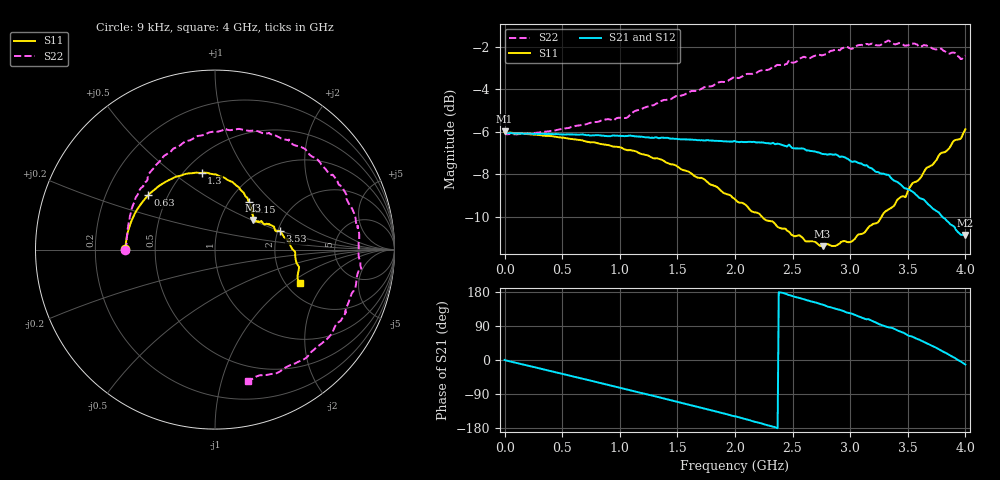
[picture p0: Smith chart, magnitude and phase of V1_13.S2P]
! ZVRE, 3.40
! symbol freq-unit parameter-type data-format keyword impedance-ohm
#  HZ  S  RI  R  50
! freq  reS11  imS11  reS21  imS21  reS12  imS12  reS22  imS22
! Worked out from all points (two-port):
!   401 points, 9 kHz to 4 GHz, reference 50 ohm
!   highest |S21| = -5.99 dB at 9 kHz (marker M1); lowest = -10.9 dB at 4 GHz (marker M2)
!   |S21| within 3 dB of the highest: start of sweep to 3.575 GHz
!   lowest |S11| = -11.4 dB at 2.76 GHz (marker M3), VSWR 1.74, Z = 71.5 + j25.6 ohm
!   |S11| at or under -10 dB: 2.232 GHz to 3.273 GHz (1.041 GHz wide, 37.8 % of centre)
!   |S22| runs from -6.1 to -1.7 dB; largest |S21 - S12| = 0.016
!   S11 on the Smith chart (normalised r, x): 9 kHz: 0.33, +0.00; 630 MHz: 0.39, +0.31; 1.3 GHz: 0.61, +0.64; 2.15 GHz: 1.23, +0.73; 3.53 GHz: 2.05, +0.49; 4 GHz: 2.38, -1.19
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9000  -0.5 0.000947  0.5017 0.000447  0.5023 -0.00206  -0.5005 -0.000708
3.200083e8  -0.462 0.1679  0.4545 -0.1973  0.4581 -0.195  -0.4859 0.1174
6.300076e8  -0.3717 0.3036  0.3422 -0.3549  0.3468 -0.3548  -0.4617 0.234
6.700075e8  -0.3578 0.3168  0.324 -0.3722  0.3293 -0.3707  -0.4564 0.249
9.800068e8  -0.2258 0.4025  0.1552 -0.4648  0.1595 -0.4665  -0.3957 0.3674
1.300006e9  -0.0742 0.4269  -0.0452 -0.4829  -0.0419 -0.485  -0.3102 0.4896
1.340006e9  -0.0551 0.4286  -0.0694 -0.4787  -0.0677 -0.4825  -0.2944 0.507
1.640005e9  0.0671 0.3897  -0.2455 -0.4118  -0.2439 -0.4145  -0.1577 0.6049
2.000004e9  0.1666 0.3046  -0.4064 -0.248  -0.4057 -0.2506  0.0617 0.6722
2.150004e9  0.1896 0.2636  -0.4486 -0.1525  -0.4477 -0.1585  0.1712 0.6642
2.390004e9  0.2077 0.2126  -0.4679 0.0135  -0.4679 0.00648  0.3433 0.6322
2.670003e9  0.2162 0.1723  -0.4055 0.1975  -0.4118 0.1908  0.5464 0.5162
2.760003e9  0.2121 0.1658  -0.3696 0.2462  -0.3777 0.2416  0.5959 0.4697
2.910002e9  0.2241 0.1562  -0.2939 0.3232  -0.2962 0.3289  0.6892 0.3631
3.070002e9  0.2408 0.1557  -0.181 0.3826  -0.183 0.3903  0.7746 0.2043
3.180002e9  0.2558 0.1589  -0.105 0.3979  -0.1082 0.4034  0.8011 0.1011
3.290002e9  0.2876 0.1446  -0.0035 0.399  -0.0113 0.4056  0.8103 -0.0692
3.340001e9  0.2983 0.1395  0.0293 0.3938  0.0315 0.3994  0.8132 -0.1064
3.530001e9  0.3608 0.1036  0.1684 0.3218  0.1713 0.3285  0.7287 -0.3475
3.670001e9  0.4098 0.0515  0.2472 0.2327  0.2528 0.236  0.6235 -0.4988
3.79e9  0.4462 -0.0147  0.2879 0.1343  0.2952 0.1334  0.4923 -0.6128
4e9  0.4728 -0.185  0.2799 -0.0595  0.2771 -0.0654  0.185 -0.7342
